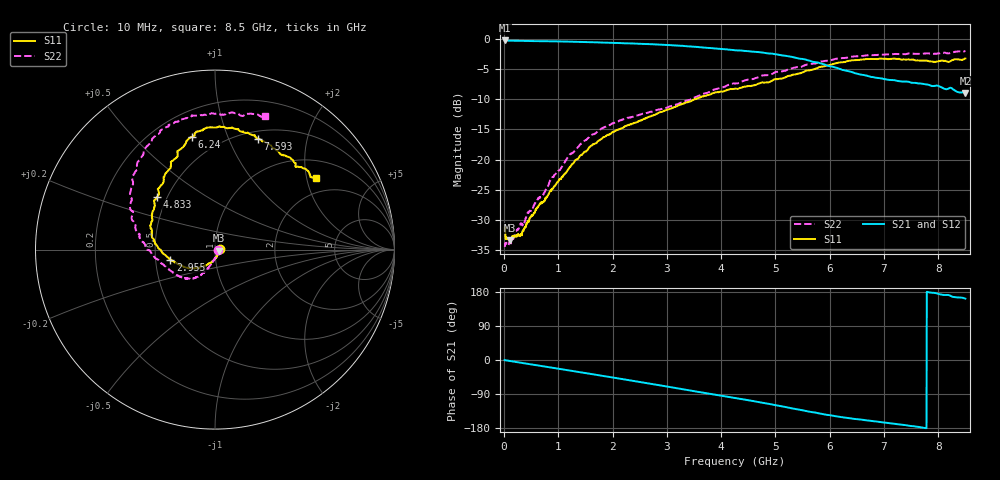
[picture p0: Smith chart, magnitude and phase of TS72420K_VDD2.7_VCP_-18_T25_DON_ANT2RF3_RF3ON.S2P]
!Agilent Technologies,E5071C,MY46417908,A.11.23
!Date: Thu Oct 03 16:41:26 2019
!Data & Calibration Information:
!Freq	S11:SOLT2(ON)	S21:SOLT2(ON)	S12:SOLT2(ON)	S22:SOLT2(ON)
!PortZ  Port1:50+j0  Port2:50+j0
!Above PortZ is port z conversion or system Z0 setting when saving the data.
!When reading, reference impedance value at option line is always used.
# Hz S dB R 50
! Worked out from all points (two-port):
!   1601 points, 10 MHz to 8.5 GHz, reference 50 ohm
!   highest |S21| = -0.26 dB at 10 MHz (marker M1); lowest = -8.9 dB at 8.5 GHz (marker M2)
!   |S21| within 3 dB of the highest: start of sweep to 5.435 GHz
!   lowest |S11| = -33.3 dB at 100.2 MHz (marker M3), VSWR 1.04, Z = 52.1 - j0.688 ohm
!   |S11| at or under -10 dB: start of sweep to 3.509 GHz
!   |S22| runs from -34.3 to -2.0 dB; largest |S21 - S12| = 0.0059
!   S11 on the Smith chart (normalised r, x): 10 MHz: 1.05, +0.01; 2.955 GHz: 0.60, -0.07; 4.833 GHz: 0.44, +0.32; 6.24 GHz: 0.35, +0.75; 7.593 GHz: 0.58, +1.29; 8.5 GHz: 1.50, +2.27
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1e7  -31.79 5.9  -0.26 -0.3  -0.24 -0.3  -34.26 -7.9
1.002062e8  -33.32 -17.8  -0.29 -2.4  -0.28 -2.5  -33.58 -23.3
3.177625e8  -32.39 -47.1  -0.33 -7.4  -0.31 -7.5  -30.54 -53.6
6.361375e8  -27.70 -78.6  -0.37 -14.6  -0.37 -14.7  -26.35 -89.2
7.210375e8  -26.99 -82.6  -0.38 -16.6  -0.38 -16.6  -25.82 -92.9
1.187988e9  -21.50 -113.7  -0.45 -27.3  -0.45 -27.3  -19.45 -109.4
1.426769e9  -19.24 -123.4  -0.51 -32.8  -0.52 -32.8  -17.33 -115.1
1.607181e9  -17.69 -130.4  -0.55 -37.0  -0.56 -37.0  -15.91 -118.5
2.015762e9  -15.41 -141.9  -0.65 -46.5  -0.65 -46.5  -13.96 -126.8
2.843538e9  -12.28 -164.6  -0.94 -66.2  -0.93 -66.3  -11.72 -148.1
2.954969e9  -11.89 -167.3  -0.99 -68.9  -0.98 -69.0  -11.48 -151.7
3.565188e9  -9.84 176.4  -1.34 -83.8  -1.32 -83.8  -9.51 -171.8
4.255e9  -8.24 156.8  -1.88 -100.2  -1.85 -100.1  -7.39 169.5
4.833381e9  -7.20 137.7  -2.38 -114.7  -2.34 -114.7  -6.01 156.1
5.31625e9  -5.94 123.3  -3.02 -127.9  -2.98 -127.8  -4.84 145.0
5.671769e9  -5.12 113.1  -3.75 -137.6  -3.73 -137.4  -4.14 135.0
6.239538e9  -3.87 101.5  -5.14 -151.0  -5.13 -150.9  -3.16 121.4
6.685262e9  -3.34 93.8  -6.10 -159.5  -6.08 -159.4  -2.72 113.9
7.088538e9  -3.34 83.7  -6.79 -166.5  -6.73 -165.9  -2.57 106.7
7.592631e9  -3.57 68.8  -7.30 -175.9  -7.35 -175.4  -2.46 96.3
8.102031e9  -3.65 48.0  -8.24 171.5  -8.30 171.3  -2.29 81.3
8.5e9  -3.24 35.4  -8.95 161.9  -8.96 161.7  -1.99 69.5
